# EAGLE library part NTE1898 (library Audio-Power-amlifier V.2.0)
Dual Audio Power Amp, 5.8W (22W BTL)
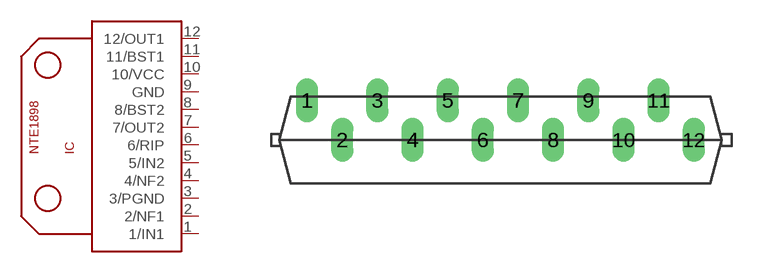
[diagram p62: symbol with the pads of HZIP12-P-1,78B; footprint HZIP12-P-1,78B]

Designator prefix IC

## NTE1898  [HZIP12-P-1,78B]
1  1/IN1  in
2  2/NF1
3  3/PGND  pwr
4  4/NF2
5  5/IN2  in
6  6/RIP
7  7/OUT2  out
8  8/BST2
9  GND  pwr
10  10/VCC  pwr
11  11/BST1
12  12/OUT1  out

## Footprint HZIP12-P-1,78B (pad centres in mm)
drill 0.6 pad 1.016 long: 1 -9.779,2; 2 -8.001,0; 3 -6.223,2; 4 -4.445,0; 5 -2.667,2; 6 -0.889,0; 7 0.889,2; 8 2.667,0; 9 4.445,2; 10 6.223,0; 11 8.001,2; 12 9.779,0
